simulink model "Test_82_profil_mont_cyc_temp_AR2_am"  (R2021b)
settings: Solver=FixedStepAuto  StartTime=0.0  StopTime=60*60*2
undefined symbols (not defined in the file): Ion, Lithium, Pe
libraries: fl_lib x31, nesl_utility x24, sdl_lib x11, simulink x5, simulink_extras x2, spsBatteryLib x1, spsCurrentVoltageSimscapeInterfaceLib x1, slpidlib x1, spspowerguiLib x1
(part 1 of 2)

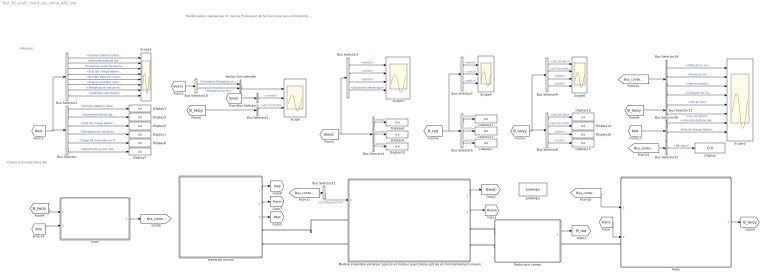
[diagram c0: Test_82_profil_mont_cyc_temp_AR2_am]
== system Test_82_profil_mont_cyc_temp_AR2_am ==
  note: Chaine d'énergie Twizy 80
  note: Modélisation réalisée par M. Garcia Professeur de S2I au lycée Louis Armand de Nogent sur Marne
  note: Mesures
  Batteries lithium : Subsystem  mask{Ubat_n=54, Qbat_n=105, Soc_init=100, Soc_min=10, T_amb=35, T_init=15, Nb_cycles=1000, Nb_charge_mensuelle=20, Nb_mois=25}
      mask prompts: Ubat_n "Tension nominale batterie en V"; Qbat_n "Capacité nominale en A.h"; Soc_init "Etat de charge initial"; Soc_min "Seuil minimum en %"; T_amb "Température ambiante extérieure en °C"; T_init "Température initiale du bloc batteries en °C"; Nb_cycles "Durée de vie batterie en nombre de cycles"; Nb_charge_mensuelle "Nombre de recharges mensuelles"; Nb_mois "Nombre de mois d'utilisation"
  Bus Selector : BusSelector  OutputSignals=tension batterie ubat(t),intensité batterie ibat(t),Etat de charge batterie soc(t) en %,Température cellule en °C,Capacité maximale en Ah,Nombre de cycles utilisés
  Bus Selector1 : BusSelector  OutputSignals=nm(t)
  Bus Selector10 : BusSelector  OutputSignals=Consigne fréquence en Hz,fréquence en Hz
  Bus Selector11 : BusSelector  OutputSignals=Consigne en %
  Bus Selector12 : BusSelector  OutputSignals=Nb_tour
  Bus Selector13 : BusSelector  OutputSignals=d(t) en km,v(t) en km/h
  Bus Selector14 : BusSelector  OutputSignals=Altitude en m,Pente en %,Vent en km/h,Consigne en %
  Bus Selector16 : BusSelector  OutputSignals=intensité batterie ibat(t),Etat de charge batterie soc(t) en %
  Bus Selector2 : BusSelector  OutputSignals=tension batterie ubat(t),intensité batterie ibat(t),Puissance consommée batterie pbat(t) en W,Etat de charge batterie soc(t) en %,Energie batterie consommée wbat_cons(t) en Wh,Energie batterie restante wbat_rest(t) en Wh,Température cellule en °C,Quadrant électrique
  Bus Selector3 : BusSelector  OutputSignals=v(t) en km/h
  Bus Selector4 : BusSelector  OutputSignals=nm(t),cm(t),pm(t)
  Bus Selector5 : BusSelector  OutputSignals=wm(t),cm(t),pm(t),Quadrant mécanique
  Bus Selector6 : BusSelector  OutputSignals=nr(t),cr(t),pr(t)
  Bus Selector7 : BusSelector  OutputSignals=wr(t),cr(t),pr(t)
  Bus Selector8 : BusSelector  OutputSignals=d(t) en km,v(t) en km/h,fm(t),pr(t)
  Bus Selector9 : BusSelector  OutputSignals=d(t) en km,v(t) en km/h,fm(t),pr(t)
  Display{,1..16} (17 alike) : Display
  Modele ensemble variateur Sevcon et moteur asynchrone Letrika en fonctionnement moyen : Subsystem  mask{Vbn=52, Tn=57, Nn=2100, fn=70, rend_mot=92, Jm=0.006, f_max_av=276, f_max_ar=41.7, rend_var=96, kp_n=1, ki_n=0.01, pas=0.1}
      mask prompts: Vbn "Tension bobinage nominale moteur en V"; Tn "Couple nominal en N.m"; Nn "Vitesse nominale moteur en tr/min"; fn "fréquence nominale moteur en Hz"; rend_mot "Rendement moteur en %"; Jm "Moment d'inertie moteur en kg.m²"; f_max_av "Fréquence maximale autorisée en marche avant en hz"; f_max_ar "Fréquence maximale autorisée en marche arrière en hz"; rend_var "Rendement variateur en %"; kp_n "Gain correcteur proportionnel"; ki_n "Gain correcteur intégral"; pas "Réglage pas solveur simscape"
  Profil : Subsystem  mask{Altitude_Pt_dep=307, Nb_portion=36, Pe_P=[4.2;6.7;5.6;5.9;6.8;7.2;6.5;6.1;7.4;3.7;3.6;8.4;7.2;8.4;6.6;4.2;3.9;0;-3.9;-4.2;-6.6;-8.4;-7.2;-8.4;-3.6;-3.7;-7.4;-6.1;-6.5;-7.2;-6.8;-5.9;-5.6;-6.7;-4.2;0], L_P=[1000;1000;1000;1000;1000;1000;1000;1000;1000;1000;1000;1000;1000;1000;1000;1000;400;2000;400;1000;1000;1000;1000;1000;1000;1000;1000;1000;1000;1000;1000;1000;1000;1000;1000;2000], Co_P=[50;50;50;50;50;50;50;50;50;50;50;50;50;50;50;50;50;25;60;60;60;60;60;60;60;60;60;60;60;60;60;60;60;60;60;25], Ve_P=[0;0;0;0;0;0;0;0;0;0;0;0;0;0;0;0;0;0;0;0;0;0;0;0;0;0;0;0;0;0;0;0;0;0;0;0], Nb_tour_max=2}
      mask prompts: Altitude_Pt_dep "Altitude du point de départ en m"; Nb_portion "Nombre de portion du circuit"; Pe_P "Pente des différentes portions en %"; L_P "Longueur des différentes portions en m"; Co_P "Consigne vitesse sur les différentes portions en %"; Ve_P "Vitesse du vent sur les différentes portions en km/h"; Nb_tour_max "Nombre de tour de circuit à parcourir"
  Reducteur comex : Subsystem  mask{ratio=(82*55)/(17*26), rend_red=96}
      mask prompts: ratio "Rapport de réduction"; rend_red "Rendement moyen transmission en %"
  Scope : Scope  NumInputPorts=3
  Scope1 : Scope  NumInputPorts=8
  Scope2 : Scope  NumInputPorts=8
  Scope3 : Scope  NumInputPorts=4
  Scope4 : Scope  NumInputPorts=3
  Scope5 : Scope  NumInputPorts=4
  Twizy : Subsystem  mask{n=2, a=733, b=955, h=900, S=1.33, Cx=0.64, M_twizy=403, M_cond=80, M_pass=0, M_Batt=71, t_jantes_av=13, l_pneu_av=125, h_broul_av=80, Prav=2.5, t_jantes_ar=13, l_pneu_ar=145, h_broul_ar=80, Prar=2.5}
      mask prompts: n "Nombre de roue par axe"; a "Distance entre position conducteur et l'axe de la roue avant en mm"; b "Distance entre position conducteur et l'axe de la roue arrière en mm"; h "Hauteur du centre de gravité passager en mm"; S "Surface frontale en m²"; Cx "Coefficient de trainée"; M_twizy "Masse twizy à vide en kg"; M_cond "Masse conducteur en kg"; M_pass "Masse passagers en kg"; M_Batt "Masse batteries en kg"; t_jantes_av "Taille jante en pouces"; l_pneu_av "Largeur en mm"; h_broul_av "Hauteur bande de roulement en %"; Prav "Pression pneus avant en bar"; t_jantes_ar "Taille jante en pouces"; l_pneu_ar "Largeur en mm"; h_broul_ar "Hauteur bande de roulement en %"; Prar "Pression pneus arrière en bar"
  Vector Concatenate : Concatenate
  powergui : spspowerguiLib/powergui  Priority=1  SimulationMode=Discrete  SampleTime=1  frequency=60  Iterations=50  frequencyindice=0  Pbase=100e6  ErrMax=1e-4  UnitsV=kV  UnitsW=MW  buscounter=0  FunctionMessages=off  echomessages=off  EnableUseOfTLC=off  CurrentSourceSwitches=off  DisableSnubberDevices=off  DisableRonSwitches=off  DisableVfSwitches=off  DisplayEquations=off  AutomaticDiscreteSolvers=off  SolverType=Tustin/Backward Euler (TBE)  Interpol=off  ExternalGateDelay=off  methode=off  Ts=100  x0status=blocks  SPID=on  SwTol=0  HookPort=off  NonlinearTolerance=1e-4  nMaxIteration=100  ContinueOnMaxIteration=off  RestoreLinks=warning  ResistiveCurrentMeasurement=off  Frange=[0:2:500]  Ylog=off  Xlog=on  ShowGrid=off  save=off  variable=ZData  structure=0  ZoomFFT=off  StartTime=0.0  cycles=1  DisplayStyle=1  fundamental=60  FreqAxis=off  MaxFrequency=1000  frequencyindicesteady=1  RmsSteady=1  display=off
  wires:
  Reducteur comex/1(Bus) -> [B_red]
  Twizy/1(Bus) -> [B_twizy]
  Modele ensemble variateur Sevcon et moteur asynchrone Letrika en fonctionnement moyen/1(Bus) -> [Bmot]
  [Freins] -> Twizy/2(Forces freinages avant et arrières)
  Modele ensemble variateur Sevcon et moteur asynchrone Letrika en fonctionnement moyen/2(Bus1) -> [Bvaria]
  Bus Selector11/1 -> Modele ensemble variateur Sevcon et moteur asynchrone Letrika en fonctionnement moyen/1(Consigne Accélérateur en %)  "<Consigne en %>"
  [B_twizy] -> Profil/1(Bus_Twizy)
  Profil/1(Contexte) -> [Bus_contexte]
  [Bus_contexte] -> Bus Selector11/1
  [Bus_contexte] -> Twizy/1(Contexte)
  Batteries lithium/1(Stop) -> [Stop]
  Batteries lithium/3(Bus batterie) -> [Bbat]
  Batteries lithium/2(Freinage) -> [Freins]
  [Stop] -> Profil/2(Stop)
  Bus Selector12/1 -> Display/1  "<Nb_tour>"
  [B_twizy] -> Bus Selector13/1
  [Bbat] -> Bus Selector16/1
  [Bvaria] -> Bus Selector10/1
  Bus Selector8/1 -> Display13/1  "<d(t) en km>"
  Bus Selector2/3 -> Scope1/3  "<Puissance consommée batterie pbat(t) en W>"
  Bus Selector/5 -> Display6/1  "<Capacité maximale en Ah>"
  [Bmot] -> Bus Selector4/1, Bus Selector5/1
  Bus Selector6/2 -> Display12/1  "<cr(t)>"
  Bus Selector6/1 -> Display11/1  "<nr(t)>"
  Bus Selector4/1 -> Display8/1  "<nm(t)>"
  Bus Selector9/3 -> Scope5/3  "<fm(t)>"
  Bus Selector5/3 -> Scope3/3  "<pm(t)>"
  Bus Selector/3 -> Display5/1  "<Etat de charge batterie soc(t) en %>"
  Bus Selector14/3 -> Scope2/3  "<Vent en km/h>"
  Bus Selector13/2 -> Scope2/6  "<v(t) en km/h>"
  [Bbat] -> Bus Selector2/1, Bus Selector/1
  Bus Selector2/8 -> Scope1/8  "<Quadrant électrique>"
  [B_twizy] -> Bus Selector3/1
  Bus Selector7/2 -> Scope4/2  "<cr(t)>"
  Bus Selector7/1 -> Scope4/1  "<wr(t)>"
  Bus Selector1/1 -> Scope/2  "<nm(t)>"
  Bus Selector7/3 -> Scope4/3  "<pr(t)>"
  Bus Selector/1 -> Display3/1  "<tension batterie ubat(t)>"
  Bus Selector2/1 -> Scope1/1  "<tension batterie ubat(t)>"
  Bus Selector/4 -> Display1/1  "<Température cellule en °C>"
  Bus Selector/2 -> Display4/1  "<intensité batterie ibat(t)>"
  Bus Selector14/2 -> Scope2/2  "<Pente en %>"
  Bus Selector5/1 -> Scope3/1  "<wm(t)>"
  Bus Selector14/4 -> Scope2/4  "<Consigne en %>"
  Bus Selector4/2 -> Display9/1  "<cm(t)>"
  Bus Selector2/5 -> Scope1/5  "<Energie batterie consommée wbat_cons(t) en Wh>"
  [B_twizy] -> Bus Selector9/1, Bus Selector8/1
  Bus Selector2/2 -> Scope1/2  "<intensité batterie ibat(t)>"
  Bus Selector10/2 -> Vector Concatenate/2  "<fréquence en Hz>"
  Bus Selector13/1 -> Scope2/5  "<d(t) en km>"
  Bus Selector/6 -> Display7/1  "<Nombre de cycles utilisés>"
  Bus Selector9/4 -> Scope5/4  "<pr(t)>"
  Bus Selector10/1 -> Vector Concatenate/1  "<Consigne fréquence en Hz>"
  Bus Selector14/1 -> Scope2/1  "<Altitude en m>"
  Bus Selector9/2 -> Scope5/2  "<v(t) en km/h>"
  Bus Selector16/2 -> Scope2/8  "<Etat de charge batterie soc(t) en %>"
  Bus Selector9/1 -> Scope5/1  "<d(t) en km>"
  Bus Selector5/2 -> Scope3/2  "<cm(t)>"
  Bus Selector5/4 -> Scope3/4  "<Quadrant mécanique>"
  [Bmot] -> Bus Selector1/1
  Bus Selector8/2 -> Display14/1  "<v(t) en km/h>"
  Bus Selector2/6 -> Scope1/6  "<Energie batterie restante wbat_rest(t) en Wh>"
  Bus Selector8/3 -> Display16/1  "<fm(t)>"
  Bus Selector3/1 -> Scope/3  "<v(t) en km/h>"
  Bus Selector6/3 -> Display2/1  "<pr(t)>"
  [Bus_contexte] -> Bus Selector14/1
  Bus Selector4/3 -> Display10/1  "<pm(t)>"
  Vector Concatenate/1 -> Scope/1
  Bus Selector8/4 -> Display15/1  "<pr(t)>"
  Bus Selector16/1 -> Scope2/7  "<intensité batterie ibat(t)>"
  Bus Selector2/7 -> Scope1/7  "<Température cellule en °C>"
  [B_red] -> Bus Selector7/1, Bus Selector6/1
  Bus Selector2/4 -> Scope1/4  "<Etat de charge batterie soc(t) en %>"
  [Bus_contexte] -> Bus Selector12/1
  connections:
  Reducteur comex/RConn1 -- Twizy/LConn1
  Reducteur comex/LConn2 -- Modele ensemble variateur Sevcon et moteur asynchrone Letrika en fonctionnement moyen/RConn2
  Reducteur comex/LConn1 -- Modele ensemble variateur Sevcon et moteur asynchrone Letrika en fonctionnement moyen/RConn1
  Modele ensemble variateur Sevcon et moteur asynchrone Letrika en fonctionnement moyen/LConn2 -- Batteries lithium/RConn2
  Modele ensemble variateur Sevcon et moteur asynchrone Letrika en fonctionnement moyen/LConn1 -- Batteries lithium/RConn1

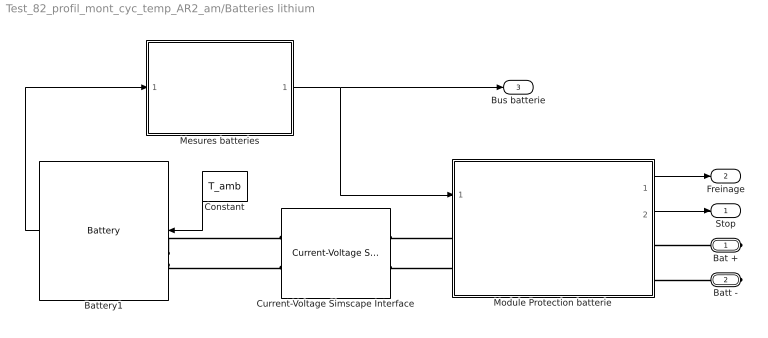
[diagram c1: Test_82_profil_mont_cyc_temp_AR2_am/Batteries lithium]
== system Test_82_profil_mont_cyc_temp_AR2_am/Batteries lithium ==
  Battery1 : spsBatteryLib/Battery  BatType=Lithium-Ion  ShowTempParam=on  ThermalPreset=no  ShowAgeParam=on  NomV=Ubat_n  NomQ=Qbat_n  SOC=Soc_init  Batt_Tr=30  PresetModel=on  MaxQ=105  MinV=40.5  FullV=62.8553  Dis_rate=45.6522  R=0.0051429  Normal_OP=94.9565  expZone="[58.3408       5.1587]"  current=[100 150 200]  Units=Time  Tci=T_init  NomT=25  T2=0  MaxQ2=Qbat_n/1.1517  FullV2=1.1933*Ubat_n  Normal_OP2=Ubat_n/1.1576  expZone2=[1.1338*Ubat_n Qbat_n/61]  Rca=0.06  ti=1000  Dp=0  Neq0=Nb_charge_mensuelle*Nb_mois  Tsim=30  Ta1=23  Qeol=0.9*Qbat_n  Reol=0.0126*1.2  Char_age=[0.38*Qbat_n, 0.495*Qbat_n]  Dis_age=[0.38*Qbat_n, 2*Qbat_n]  N1=Nb_cycles  N2=7*Nb_cycles  N3=Nb_cycles/1.5  N4=Nb_cycles*0.9733  Ta2=45  N5=Nb_cycles*0.655
  Constant : Constant  Value=T_amb
  Current-Voltage Simscape Interface : spsCurrentVoltageSimscapeInterfaceLib/Current-Voltage Simscape Interface  DFT=off  FMode=Unit delay (discrete)  T=1e-6  Ts=-1  i0=0  v0=52  Sd=Simscape side  Measurements=off
  Mesures batteries : Subsystem
  Module Protection batterie : Subsystem
  Bat + : PMIOPort  Side=Right
  Batt - : PMIOPort  Port=2  Side=Right
  Stop : Outport  VectorParamsAs1DForOutWhenUnconnected=off
  Freinage : Outport  Port=2  VectorParamsAs1DForOutWhenUnconnected=off
  Bus batterie : Outport  Port=3  VectorParamsAs1DForOutWhenUnconnected=off
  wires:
  Battery1/1 -> Mesures batteries/1(Bus batteries)
  Mesures batteries/1(Bus_ batteries) -> Module Protection batterie/1(Bus batterie), Bus batterie/1
  Module Protection batterie/1(Freinage) -> Freinage/1
  Module Protection batterie/2(Stop) -> Stop/1
  Constant/1 -> Battery1/1
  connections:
  Battery1/LConn2 -- Current-Voltage Simscape Interface/LConn2
  Battery1/LConn1 -- Current-Voltage Simscape Interface/LConn1
  Module Protection batterie/RConn2 -- Batt -/RConn1
  Module Protection batterie/RConn1 -- Bat +/RConn1
  Module Protection batterie/LConn1 -- Current-Voltage Simscape Interface/RConn1
  Module Protection batterie/LConn2 -- Current-Voltage Simscape Interface/RConn2

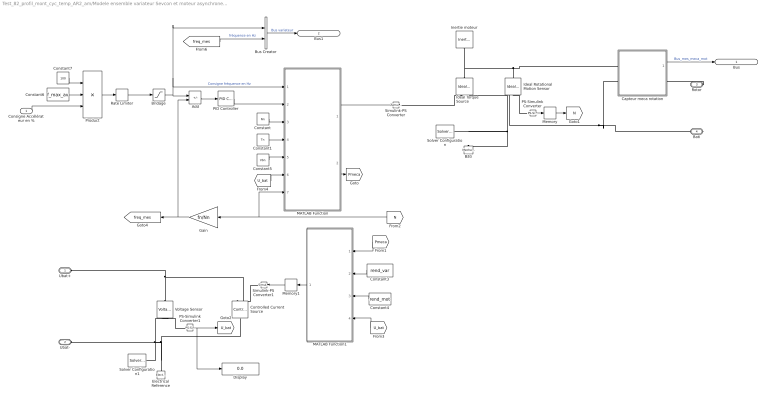
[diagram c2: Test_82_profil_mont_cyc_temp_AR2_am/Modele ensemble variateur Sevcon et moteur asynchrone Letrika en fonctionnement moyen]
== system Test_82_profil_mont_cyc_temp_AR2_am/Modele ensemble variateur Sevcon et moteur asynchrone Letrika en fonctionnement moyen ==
  Consigne Accélérateur en % : Inport
  Add : Sum  Inputs=+-
  Bridage : Saturate  UpperLimit=f_max_av  LowerLimit=-f_max_ar
  Bus Creator : BusCreator  Inputs=2
  Bâti : fl_lib/Mechanical/Rotational Elements/Mechanical Rotational Reference
  Capteur meca rotation : Subsystem
  Constant : Constant  Value=Nn
  Constant1 : Constant  Value=Tn
  Constant3 : Constant  Value=rend_var
  Constant4 : Constant  Value=rend_mot
  Constant5 : Constant  Value=Vbn
  Constant6 : Constant  Value=f_max_av
  Constant7 : Constant  Value=100
  Controlled Current Source : fl_lib/Electrical/Electrical Sources/Controlled Current Source
  Display : Display
  Electrical Reference : fl_lib/Electrical/Electrical Elements/Electrical Reference
  Gain : Gain  Gain=fn/Nn
  Ideal Rotational Motion Sensor : fl_lib/Mechanical/Mechanical Sensors/Ideal Rotational Motion Sensor  wrap_angle=simscape.enum.onoff.off  offset=0 rad
  Ideal Torque Source : fl_lib/Mechanical/Mechanical Sources/Ideal Torque Source
  Inertie moteur : fl_lib/Mechanical/Rotational Elements/Inertia  inertia=Jm kg*m^2  num_ports=foundation.enum.numPorts2.one  w_specify=off  w_priority=High  w=0 rad/s  w_nominal_specify=off  w_nominal_unit=rad/s  w_nominal_value=1  t_specify=off  t_priority=None  t=0 N*m  t_nominal_specify=off  t_nominal_unit=N*m  t_nominal_value=1
  MATLAB Function : MATLAB Function  TreatAsAtomicUnit=on
  MATLAB Function1 : MATLAB Function  TreatAsAtomicUnit=on
  Memory : Memory
  Memory1 : Memory
  PID Controller : slpidlib/PID Controller  Controller=PID  Form=Parallel  TimeDomain=Continuous-time  UseExternalTs=off  SampleTime=-1  IntegratorMethod=Forward Euler  FilterMethod=Forward Euler  ControllerParametersSource=internal  P=kp_n  I=ki_n  D=0  UseFilter=on  N=100  TunerSelectOption=Transfer Function Based (PID Tuner App)  InitialConditionSource=internal  InitialConditionForIntegrator=0  InitialConditionForFilter=0  DifferentiatorICPrevScaledInput=0  ExternalReset=none  TrackingMode=off  Kt=1  LimitOutput=off  SatLimitsSource=internal  UpperSaturationLimit=inf  LowerSaturationLimit=-inf  LinearizeAsGain=on  AntiWindupMode=none  Kb=1  POutMin=[]  POutMax=[]  IOutMin=[]  IOutMax=[]  DOutMin=[]  DOutMax=[]  NOutMin=[]  NOutMax=[]  SumOutMin=[]  SumOutMax=[]  SaturationOutMin=[]  SaturationOutMax=[]  PParamMin=[]  PParamMax=[]  IParamMin=[]  IParamMax=[]  DParamMin=[]  DParamMax=[]  NParamMin=[]  NParamMax=[]  KbParamMin=[]  KbParamMax=[]  KtParamMin=[]  KtParamMax=[]  KbOutMin=[]  KbOutMax=[]  KtOutMin=[]  KtOutMax=[]  IntegratorOutMin=[]  IntegratorOutMax=[]  FilterOutMin=[]  FilterOutMax=[]  SumI1OutMin=[]  SumI1OutMax=[]  SumI2OutMin=[]  SumI2OutMax=[]  SumI3OutMin=[]  SumI3OutMax=[]  SumI4OutMin=[]  SumI4OutMax=[]  SumDOutMin=[]  SumDOutMax=[]  DifferentiatorOutMin=[]  DifferentiatorOutMax=[]  FilterDiffOutCoefMin=[]  FilterDiffOutCoefMax=[]  ReciprocalOutMin=[]  ReciprocalOutMax=[]  SumDenOutMin=[]  SumDenOutMax=[]  SumNumOutMin=[]  SumNumOutMax=[]  DivideOutMin=[]  DivideOutMax=[]  UdiffTsProdOutMin=[]  UdiffTsProdOutMax=[]  NTsProdOutMin=[]  NTsProdOutMax=[]  UintegralTsProdOutMin=[]  UintegralTsProdOutMax=[]  UngainTsProdOutMin=[]  UngainTsProdOutMax=[]  IntegratorContinuousStateAttributes=''  IntegratorStateMustResolveToSignalObject=off  IntegratorRTWStateStorageClass=Auto  FilterContinuousStateAttributes=''  FilterStateMustResolveToSignalObject=off  FilterRTWStateStorageClass=Auto  ParallelPVariant=InternalParameters  IdealPVariant=Disabled  IVariant=InternalParameters  DVariant=InternalParameters  IntegratorVariant=Continuous  SatVariant=Disabled  AWVariant=Passthrough  PCopyVariant=Disabled  TRVariant=Disabled  FdbkBlocksVariant=Forward  IdealPFdbkVariant=Disabled  SatFdbkVariant=Disabled  DerivativeFilterVariant=ContFilter  NVariant=InternalParameters  NCopyVariant=Disabled  FilterICVariant=InternalICsFilter  IntegratorICVariant=InternalICs  ExternalResetVariant=Disabled  TRSumVariant=Passthrough  SumFdbkVariant=Disabled  SumVariant=Sum_PID  TsampFilterVariant=InternalTs  TsampNgainVariant=Passthrough  TsampIntegralVariant=Passthrough  ExternalSaturationOutDataTypeStr=Inherit: Same as second input
  PS-Simulink Converter : nesl_utility/PS-Simulink Converter  PhysicalDomain=network_engine_domain  SubClassName=ps_output  LeftPortType=input  RightPortType=output  PseudoPeriodic=off  Frequencies=[]  Unit=rpm  AffineConversion=off
  PS-Simulink Converter1 : nesl_utility/PS-Simulink Converter  PhysicalDomain=network_engine_domain  SubClassName=ps_output  LeftPortType=input  RightPortType=output  PseudoPeriodic=off  Frequencies=[]  Unit=V  AffineConversion=off
  Product : Product  Inputs=/**
  Rate Limiter : RateLimiter  RisingSlewLimit=80  FallingSlewLimit=-inf  SampleTimeMode=inherited
  Simulink-PS Converter : nesl_utility/Simulink-PS Converter  PhysicalDomain=network_engine_domain  SubClassName=ps_input  LeftPortType=input  RightPortType=output  PseudoPeriodic=off  Frequencies=[]  NoiseDistribution=none  NoiseParameters=[]  Unit=N*m  AffineConversion=off  FilteringAndDerivatives=provide  SimscapeFilterOrder=1  InputFilterTimeConstant=0.001  UdotUserProvided=0
  Simulink-PS Converter1 : nesl_utility/Simulink-PS Converter  PhysicalDomain=network_engine_domain  SubClassName=ps_input  LeftPortType=input  RightPortType=output  PseudoPeriodic=off  Frequencies=[]  NoiseDistribution=none  NoiseParameters=[]  Unit=A  AffineConversion=off  FilteringAndDerivatives=provide  SimscapeFilterOrder=1  InputFilterTimeConstant=0.001  UdotUserProvided=0
  Solver Configuration : nesl_utility/Solver Configuration  PhysicalDomain=network_engine_domain  SubClassName=solver  LeftPortType=input  RightPortType=generic  Tones=[]  Harmonics=[]  SimulateNoise=off  Profile=off  UseLocalSampling=off  EnableSwitchedLinearOptims=on  FrequencyDomain=off  UseCCode=off  RelTol=0.001  AbsTol=1e-06  MinStep=1e-09  ToWorkspace=off  RevertToSquareIcSolve=off  NumHomotopyIterations=100  PhasorMode=off  PhasorModeNumHarmonics=1  DoDC=off  ResidualTolerance=1e-9  UseLocalSolver=on  LocalSolverChoice=NE_BACKWARD_EULER_ADVANCER  LocalSolverSampleTime=pas  DoFixedCost=on  MaxNonlinIter=3  MaxModeIter=2  ComputeImpulses=off  ImpulseIterations=2  LinearAlgebra=auto  EquationFormulation=NE_TIME_EF  DelaysMemoryBudget=1024  AutomaticFiltering=on  FilteringTimeConstant=0.001  PartitionStorageMethod=AS_NEEDED  PartitionMemoryBudget=1024  PartitionMethod=FAST
  Solver Configuration1 : nesl_utility/Solver Configuration  PhysicalDomain=network_engine_domain  SubClassName=solver  LeftPortType=input  RightPortType=generic  Tones=[]  Harmonics=[]  SimulateNoise=off  Profile=off  UseLocalSampling=off  EnableSwitchedLinearOptims=on  FrequencyDomain=off  UseCCode=off  RelTol=0.001  AbsTol=1e-06  MinStep=1e-09  ToWorkspace=off  RevertToSquareIcSolve=off  NumHomotopyIterations=100  PhasorMode=off  PhasorModeNumHarmonics=1  DoDC=off  ResidualTolerance=1e-9  UseLocalSolver=on  LocalSolverChoice=NE_BACKWARD_EULER_ADVANCER  LocalSolverSampleTime=pas  DoFixedCost=on  MaxNonlinIter=3  MaxModeIter=2  ComputeImpulses=off  ImpulseIterations=2  LinearAlgebra=auto  EquationFormulation=NE_TIME_EF  DelaysMemoryBudget=1024  AutomaticFiltering=on  FilteringTimeConstant=0.001  PartitionStorageMethod=AS_NEEDED  PartitionMemoryBudget=1024  PartitionMethod=FAST
  Voltage Sensor : fl_lib/Electrical/Electrical Sensors/Voltage Sensor
  Ubat+ : PMIOPort  Side=Left
  Ubat- : PMIOPort  Port=2  Side=Left
  Rotor : PMIOPort  Port=3  Side=Right
  Bati : PMIOPort  Port=4  Side=Right
  Bus : Outport  VectorParamsAs1DForOutWhenUnconnected=off
  Bus1 : Outport  Port=2  VectorParamsAs1DForOutWhenUnconnected=off
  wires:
  Capteur meca rotation/1(Out6) -> Bus/1  "Bus_mes_meca_mot"
  PS-Simulink Converter/1 -> Memory/1
  Constant/1 -> MATLAB Function/3(Nn)
  Constant1/1 -> MATLAB Function/4(Tn)
  [N] -> Gain/1, MATLAB Function/7(Nmes)
  Add/1 -> PID Controller/1
  PID Controller/1 -> MATLAB Function/2(T_in)
  Consigne Accélérateur en %/1 -> Product/3
  Memory/1 -> [N]
  MATLAB Function1/1(I_bat) -> Memory1/1
  MATLAB Function/2(P_meca) -> [Pmeca]
  [Pmeca] -> MATLAB Function1/1(Pmeca)
  Constant3/1 -> MATLAB Function1/2(rend_var)
  Constant4/1 -> MATLAB Function1/3(rend_mot)
  PS-Simulink Converter1/1 -> Display/1, [U_bat]
  [U_bat] -> MATLAB Function1/4(U_bat)
  [U_bat] -> MATLAB Function/6(U_bat)
  Constant5/1 -> MATLAB Function/5(Un)
  Gain/1 -> [freq_mes], Add/2
  Constant6/1 -> Product/2
  Constant7/1 -> Product/1
  Bus Creator/1 -> Bus1/1  "Bus variateur"
  Bridage/1 -> Bus Creator/1, MATLAB Function/1(Consigne_frequence), Add/1  "Consigne fréquence en Hz"
  [freq_mes] -> Bus Creator/2  "fréquence en Hz"
  Memory1/1 -> Simulink-PS Converter1/1
  MATLAB Function/1(T_out) -> Simulink-PS Converter/1
  Product/1 -> Rate Limiter/1
  Rate Limiter/1 -> Bridage/1
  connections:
  Rotor/RConn1 -- Capteur meca rotation/RConn1
  Ideal Rotational Motion Sensor/RConn1 -- Bâti/LConn1 -- Solver Configuration/RConn1 -- Ideal Torque Source/RConn2 -- Bati/RConn1 -- Capteur meca rotation/LConn2
  Ideal Torque Source/LConn1 -- Inertie moteur/LConn1 -- Capteur meca rotation/LConn1 -- Ideal Rotational Motion Sensor/LConn1
  PS-Simulink Converter/LConn1 -- Ideal Rotational Motion Sensor/RConn2
  Simulink-PS Converter/RConn1 -- Ideal Torque Source/RConn1
  Ubat-/RConn1 -- Controlled Current Source/LConn1 -- Electrical Reference/LConn1 -- Solver Configuration1/RConn1 -- Voltage Sensor/RConn2
  PS-Simulink Converter1/LConn1 -- Voltage Sensor/RConn1
  Simulink-PS Converter1/RConn1 -- Controlled Current Source/RConn1
  Voltage Sensor/LConn1 -- Ubat+/RConn1 -- Controlled Current Source/RConn2

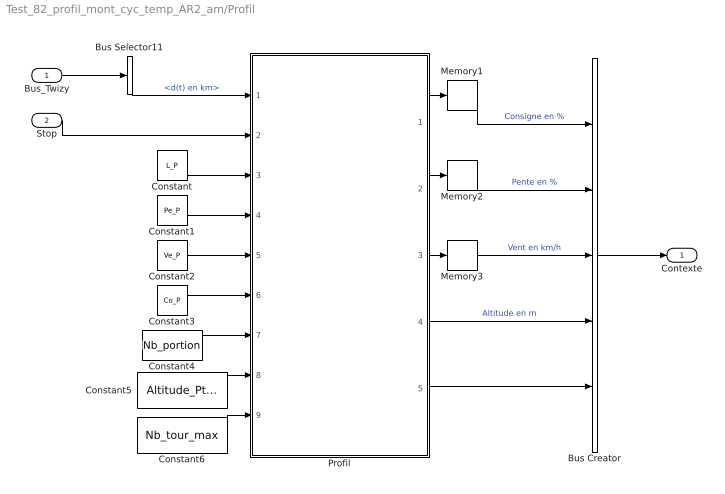
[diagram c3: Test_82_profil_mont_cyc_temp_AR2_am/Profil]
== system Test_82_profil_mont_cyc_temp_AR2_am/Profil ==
  Bus_Twizy : Inport
  Stop : Inport  Port=2
  Bus Creator : BusCreator  Inputs=5
  Bus Selector11 : BusSelector  OutputSignals=d(t) en km
  Constant : Constant  Value=L_P
  Constant1 : Constant  Value=Pe_P
  Constant2 : Constant  Value=Ve_P
  Constant3 : Constant  Value=Co_P
  Constant4 : Constant  Value=Nb_portion
  Constant5 : Constant  Value=Altitude_Pt_dep
  Constant6 : Constant  Value=Nb_tour_max
  Memory1 : Memory
  Memory2 : Memory
  Memory3 : Memory
  Profil : Stateflow chart  TreatAsAtomicUnit=on
  Contexte : Outport  VectorParamsAs1DForOutWhenUnconnected=off
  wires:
  Profil/3(Vent) -> Memory3/1
  Profil/4(Hauteur) -> Bus Creator/4  "Altitude en m"
  Constant/1 -> Profil/3(L_P)
  Constant6/1 -> Profil/9(Nb_tour_max)
  Constant5/1 -> Profil/8(Altitude_Pt_dep)
  Constant3/1 -> Profil/6(Co_P)
  Constant4/1 -> Profil/7(Nb_portion)
  Constant2/1 -> Profil/5(Ve_P)
  Bus_Twizy/1 -> Bus Selector11/1
  Constant1/1 -> Profil/4(Pe_P)
  Memory1/1 -> Bus Creator/1  "Consigne en %"
  Stop/1 -> Profil/2(Stop)
  Profil/2(Pente) -> Memory2/1
  Memory3/1 -> Bus Creator/3  "Vent en km/h"
  Memory2/1 -> Bus Creator/2  "Pente en %"
  Profil/1(Consigne_vit) -> Memory1/1
  Bus Selector11/1 -> Profil/1(position)  "<d(t) en km>"
  Bus Creator/1 -> Contexte/1
  Profil/5(Nb_tour) -> Bus Creator/5

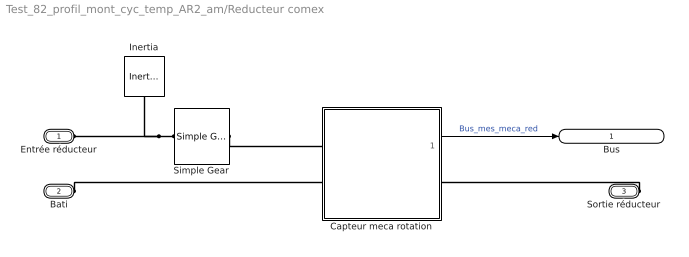
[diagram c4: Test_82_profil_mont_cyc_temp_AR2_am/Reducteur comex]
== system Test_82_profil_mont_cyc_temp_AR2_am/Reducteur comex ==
  Capteur meca rotation : Subsystem
  Inertia : fl_lib/Mechanical/Rotational Elements/Inertia  inertia=0.0725 kg*m^2  num_ports=foundation.enum.numPorts2.one  w_specify=off  w_priority=High  w=0 rad/s  w_nominal_specify=off  w_nominal_unit=rad/s  w_nominal_value=1  t_specify=off  t_priority=None  t=0 N*m  t_nominal_specify=off  t_nominal_unit=N*m  t_nominal_value=1
  Simple Gear : sdl_lib/Gears/Simple Gear  ratio=ratio  rotation_direction=3-2*(1)  friction_model=2  T_noload=0.1 N*m  T_nom=5 N*m  efficiency_nom=0.8  efficiency=rend_red/100  temperature_TLU=[280, 300, 320] K  load_TLU=[1, 5, 10] N*m  efficiency_TLU=[.95, .9, .85]  efficiency_TLU2=[.85, .8, .75; .95, .9, .85; .85, .8, .7]  w_thr=0.01 rad/s  pwr_thr=0.001 W  backlash_model=sdl.enum.backlashModel.Off  backlash_distance=1e-3 mm  x0=0 mm  r_base=0.1 m  hardstop_model=simscape.enum.hardstop.smooth  transition=1e-4 mm  backlash_stiffness=1e7 N/m  backlash_damping=1e6 N*s/m  e=0  v_tol=0.001 m/s  mu_visc=[0, 0] N*m/(rad/s)  enable_faults=0  efficiency_fault=0.05  external_fault=simscape.enum.onoff.off  temporal_fault=0  fault_time=5 s  fault_angles=pi / 12 rad  report_fault=(1)-1  thermal_mass=50 J/K  temperature_specify=off  temperature_priority=High  temperature=300 K  temperature_nominal_specify=off  temperature_nominal_unit=K  temperature_nominal_value=1  x_backlash_specify=off  x_backlash_priority=None  x_backlash=0 mm  x_backlash_nominal_specify=off  x_backlash_nominal_unit=mm  x_backlash_nominal_value=1  f_hardstop_specify=off  f_hardstop_priority=None  f_hardstop=0 N  f_hardstop_nominal_specify=off  f_hardstop_nominal_unit=N  f_hardstop_nominal_value=1  v_backlash_specify=off  v_backlash_priority=None  v_backlash=0 m/s  v_backlash_nominal_specify=off  v_backlash_nominal_unit=m/s  v_backlash_nominal_value=1
  Entrée réducteur : PMIOPort  Side=Left
  Bati : PMIOPort  Port=2  Side=Left
  Sortie réducteur : PMIOPort  Port=3  Side=Right
  Bus : Outport  VectorParamsAs1DForOutWhenUnconnected=off
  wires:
  Capteur meca rotation/1(Out6) -> Bus/1  "Bus_mes_meca_red"
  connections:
  Sortie réducteur/RConn1 -- Capteur meca rotation/RConn1
  Simple Gear/LConn1 -- Inertia/LConn1 -- Entrée réducteur/RConn1
  Bati/RConn1 -- Capteur meca rotation/LConn2
  Simple Gear/RConn1 -- Capteur meca rotation/LConn1

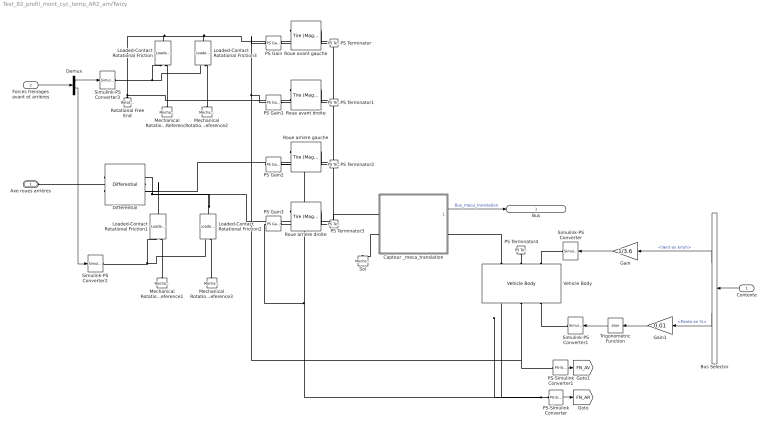
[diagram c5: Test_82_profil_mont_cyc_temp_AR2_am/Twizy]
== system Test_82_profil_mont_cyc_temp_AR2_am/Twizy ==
  Contexte : Inport
  Forces freinages avant et arrières : Inport  Port=2
  Bus Selector : BusSelector  OutputSignals=Vent en km/h,Pente en %
  Capteur _meca_translation : Subsystem
  Demux : Demux  Outputs=2
  Differential : sdl_lib/Gears/Differential  driveshaft_location=2  cd_ratio=1  friction_model=1  efficiency=[ 0.85 0.92 ]  temperature_TLU=[280, 300, 320] K  efficiency_ss_TLU=[.95, .9, .85]  efficiency_cd_TLU=[.95, .9, .85]  pwr_thr=[.001, .001] W  mu_visc=[ 0 0 ] N*m/(rad/s)  model_inertia=1  carrier_inertia=0.2 kg*m^2  planet_inertia=0.02 kg*m^2  thermal_mass=50 J/K  T_init=300 K
  Gain : Gain  Gain=1/3.6
  Gain1 : Gain  Gain=0.01
  Loaded-Contact Rotational Friction : sdl_lib/Brakes & Detents/Rotational/Loaded-Contact Rotational Friction  geometry_model=1  r_eff=280 mm  d_o=150 mm  d_i=100 mm  friction_model=1  mu_w_vector=[ 0 0.1 0.2 0.3 0.4 0.5 1 2 5 10 100 1000 ] rad/s  temperature_TLU=[280, 300, 320] K  mu_static=0.35  mu_static_vector=[.4, .38, .36]  mu_coulomb=0.3  mu_coulomb_vector=[ 0.29 0.28 0.26 0.22 0.21 0.2 0.2 0.19 0.19 0.19 0.19 0.19 ]  mu_coulomb_temp_vector=[.3, .28, .25]  mu_coulomb_matrix=[.34, .32, .3; .3, .28, .25; .25, .2, .15]  mu_interp_method=simscape.enum.interpolation.linear  mu_extrap_method=simscape.enum.extrapolation.linear  w_tol=0.001 rad/s  force_min=1 N  mu_visc=0 N*m/(rad/s)  initial_state_locked=0  enable_faults=simscape.enum.onoff.off  fault_type=sdl.enum.clutchFault.lock  external_fault=simscape.enum.onoff.off  temporal_fault=simscape.enum.onoff.off  fault_time=5 s  report_fault=simscape.enum.assert.action.none  thermal_mass=50 kJ/K  T_init=300 K
  Loaded-Contact Rotational Friction1 : sdl_lib/Brakes & Detents/Rotational/Loaded-Contact Rotational Friction  geometry_model=1  r_eff=280 mm  d_o=150 mm  d_i=100 mm  friction_model=1  mu_w_vector=[ 0 0.1 0.2 0.3 0.4 0.5 1 2 5 10 100 1000 ] rad/s  temperature_TLU=[280, 300, 320] K  mu_static=0.35  mu_static_vector=[.4, .38, .36]  mu_coulomb=0.3  mu_coulomb_vector=[ 0.29 0.28 0.26 0.22 0.21 0.2 0.2 0.19 0.19 0.19 0.19 0.19 ]  mu_coulomb_temp_vector=[.3, .28, .25]  mu_coulomb_matrix=[.34, .32, .3; .3, .28, .25; .25, .2, .15]  mu_interp_method=1  mu_extrap_method=1  w_tol=0.001 rad/s  force_min=1 N  mu_visc=0 N*m/(rad/s)  initial_state_locked=0  enable_faults=simscape.enum.onoff.off  fault_type=sdl.enum.clutchFault.lock  external_fault=simscape.enum.onoff.off  temporal_fault=simscape.enum.onoff.off  fault_time=5 s  report_fault=simscape.enum.assert.action.none  thermal_mass=50 kJ/K  T_init=300 K
  Loaded-Contact Rotational Friction2 : sdl_lib/Brakes & Detents/Rotational/Loaded-Contact Rotational Friction  geometry_model=1  r_eff=280 mm  d_o=150 mm  d_i=100 mm  friction_model=1  mu_w_vector=[ 0 0.1 0.2 0.3 0.4 0.5 1 2 5 10 100 1000 ] rad/s  temperature_TLU=[280, 300, 320] K  mu_static=0.35  mu_static_vector=[.4, .38, .36]  mu_coulomb=0.3  mu_coulomb_vector=[ 0.29 0.28 0.26 0.22 0.21 0.2 0.2 0.19 0.19 0.19 0.19 0.19 ]  mu_coulomb_temp_vector=[.3, .28, .25]  mu_coulomb_matrix=[.34, .32, .3; .3, .28, .25; .25, .2, .15]  mu_interp_method=1  mu_extrap_method=1  w_tol=0.001 rad/s  force_min=1 N  mu_visc=0 N*m/(rad/s)  initial_state_locked=0  enable_faults=simscape.enum.onoff.off  fault_type=sdl.enum.clutchFault.lock  external_fault=simscape.enum.onoff.off  temporal_fault=simscape.enum.onoff.off  fault_time=5 s  report_fault=simscape.enum.assert.action.none  thermal_mass=50 kJ/K  T_init=300 K
  Loaded-Contact Rotational Friction3 : sdl_lib/Brakes & Detents/Rotational/Loaded-Contact Rotational Friction  geometry_model=1  r_eff=280 mm  d_o=150 mm  d_i=100 mm  friction_model=1  mu_w_vector=[ 0 0.1 0.2 0.3 0.4 0.5 1 2 5 10 100 1000 ] rad/s  temperature_TLU=[280, 300, 320] K  mu_static=0.35  mu_static_vector=[.4, .38, .36]  mu_coulomb=0.3  mu_coulomb_vector=[ 0.29 0.28 0.26 0.22 0.21 0.2 0.2 0.19 0.19 0.19 0.19 0.19 ]  mu_coulomb_temp_vector=[.3, .28, .25]  mu_coulomb_matrix=[.34, .32, .3; .3, .28, .25; .25, .2, .15]  mu_interp_method=simscape.enum.interpolation.linear  mu_extrap_method=simscape.enum.extrapolation.linear  w_tol=0.001 rad/s  force_min=1 N  mu_visc=0 N*m/(rad/s)  initial_state_locked=0  enable_faults=simscape.enum.onoff.off  fault_type=sdl.enum.clutchFault.lock  external_fault=simscape.enum.onoff.off  temporal_fault=simscape.enum.onoff.off  fault_time=5 s  report_fault=simscape.enum.assert.action.none  thermal_mass=50 kJ/K  T_init=300 K
  Mechanical Rotational Reference{,1..3} (4 alike) : fl_lib/Mechanical/Rotational Elements/Mechanical Rotational Reference
  PS Gain{,1..3} (4 alike) : fl_lib/Physical Signals/Functions/PS Gain  gain=0.5
  PS Terminator{,1..4} (5 alike) : fl_lib/Physical Signals/Sinks/PS Terminator
  PS-Simulink Converter : nesl_utility/PS-Simulink Converter  PhysicalDomain=network_engine_domain  SubClassName=ps_output  LeftPortType=input  RightPortType=output  PseudoPeriodic=off  Frequencies=[]  Unit=N  AffineConversion=off
  PS-Simulink Converter1 : nesl_utility/PS-Simulink Converter  PhysicalDomain=network_engine_domain  SubClassName=ps_output  LeftPortType=input  RightPortType=output  PseudoPeriodic=off  Frequencies=[]  Unit=N  AffineConversion=off
  Rotational Free End : fl_lib/Mechanical/Rotational Elements/Rotational Free End  w_specify=off  w_priority=None  w=0 rad/s  w_nominal_specify=off  w_nominal_unit=rad/s  w_nominal_value=1
  Roue arriere droite : sdl_lib/Tires & Vehicles/Tire (Magic Formula)  parameterization=sdl.enum.magic_tire_model.constant  F_z1=3e+3 N  F_x1=3.5e+3 N  kappa1=10  B_m=10  C_m=1.9  D_m=1  E_m=0.97  fz0=4e+3 N  p_Cx=1.685  p_Dx=[ 1.21 -0.037 ]  p_Ex=[ 0.344 0.095 -0.02 0 ]  p_Kx=[ 21.51 -0.163 0.245 ]  p_Hx=[ -0.002 0.002 ]  p_Vx=[ 0 0 ]  r_e=(t_jantes_av*25.4+2*l_pneu_av*h_broul_av/100)/2 mm  model_compliance=sdl.enum.compliance.on  stiffness=1e+6 N/m  damping=1000 N/(m/s)  model_inertia=sdl.enum.model_inertia.on  inertia=0.12 kg*m^2  initial_velocity=0 rad/s  model_resistance=simscape.enum.onoff.on  resistance_model=sdl.enum.rollingResistanceParameterization.velocity  coeff=0.027*Pe  p_tire=Prar bar  alpha=-0.003  beta=0.76  coeff_a=84e-4  coeff_b=6.2e-4 s/m  coeff_c=1.6e-4 s^2/m^2  v_thr=1e-3 m/s  v_tr_thr=0.1 m/s
  Roue arriere gauche : sdl_lib/Tires & Vehicles/Tire (Magic Formula)  parameterization=sdl.enum.magic_tire_model.constant  F_z1=3e+3 N  F_x1=3.5e+3 N  kappa1=10  B_m=10  C_m=1.9  D_m=1  E_m=0.97  fz0=4e+3 N  p_Cx=1.685  p_Dx=[ 1.21 -0.037 ]  p_Ex=[ 0.344 0.095 -0.02 0 ]  p_Kx=[ 21.51 -0.163 0.245 ]  p_Hx=[ -0.002 0.002 ]  p_Vx=[ 0 0 ]  r_e=(t_jantes_av*25.4+2*l_pneu_av*h_broul_av/100)/2 mm  model_compliance=sdl.enum.compliance.on  stiffness=1e+6 N/m  damping=1000 N/(m/s)  model_inertia=sdl.enum.model_inertia.on  inertia=0.12 kg*m^2  initial_velocity=0 rad/s  model_resistance=simscape.enum.onoff.on  resistance_model=sdl.enum.rollingResistanceParameterization.velocity  coeff=0.027*Pe  p_tire=Prar bar  alpha=-0.003  beta=0.76  coeff_a=84e-4  coeff_b=6.2e-4 s/m  coeff_c=1.6e-4 s^2/m^2  v_thr=1e-3 m/s  v_tr_thr=0.1 m/s
  Roue avant droite : sdl_lib/Tires & Vehicles/Tire (Magic Formula)  parameterization=sdl.enum.magic_tire_model.constant  F_z1=3e+3 N  F_x1=3.5e+3 N  kappa1=10  B_m=10  C_m=1.9  D_m=1  E_m=0.97  fz0=4e+3 N  p_Cx=1.685  p_Dx=[ 1.21 -0.037 ]  p_Ex=[ 0.344 0.095 -0.02 0 ]  p_Kx=[ 21.51 -0.163 0.245 ]  p_Hx=[ -0.002 0.002 ]  p_Vx=[ 0 0 ]  r_e=(t_jantes_av*25.4+2*l_pneu_av*h_broul_av/100)/2 mm  model_compliance=sdl.enum.compliance.on  stiffness=1e+6 N/m  damping=1000 N/(m/s)  model_inertia=sdl.enum.model_inertia.on  inertia=0.12 kg*m^2  initial_velocity=0 rad/s  model_resistance=simscape.enum.onoff.on  resistance_model=sdl.enum.rollingResistanceParameterization.velocity  coeff=0.027*Pe  p_tire=Prav bar  alpha=-0.003  beta=0.76  coeff_a=84e-4  coeff_b=6.2e-4 s/m  coeff_c=1.6e-4 s^2/m^2  v_thr=1e-3 m/s  v_tr_thr=0.1 m/s
  Roue avant gauche : sdl_lib/Tires & Vehicles/Tire (Magic Formula)  parameterization=sdl.enum.magic_tire_model.constant  F_z1=3e+3 N  F_x1=3.5e+3 N  kappa1=10  B_m=10  C_m=1.9  D_m=1  E_m=0.97  fz0=4e+3 N  p_Cx=1.685  p_Dx=[ 1.21 -0.037 ]  p_Ex=[ 0.344 0.095 -0.02 0 ]  p_Kx=[ 21.51 -0.163 0.245 ]  p_Hx=[ -0.002 0.002 ]  p_Vx=[ 0 0 ]  r_e=(t_jantes_av*25.4+2*l_pneu_av*h_broul_av/100)/2 mm  model_compliance=sdl.enum.compliance.on  stiffness=1e+6 N/m  damping=1000 N/(m/s)  model_inertia=sdl.enum.model_inertia.on  inertia=0.12 kg*m^2  initial_velocity=0 rad/s  model_resistance=simscape.enum.onoff.on  resistance_model=sdl.enum.rollingResistanceParameterization.velocity  coeff=0.027*Pe  p_tire=Prav bar  alpha=-0.003  beta=0.76  coeff_a=84e-4  coeff_b=6.2e-4 s/m  coeff_c=1.6e-4 s^2/m^2  v_thr=1e-3 m/s  v_tr_thr=0.1 m/s
  Simulink-PS Converter : nesl_utility/Simulink-PS Converter  PhysicalDomain=network_engine_domain  SubClassName=ps_input  LeftPortType=input  RightPortType=output  PseudoPeriodic=off  Frequencies=[]  NoiseDistribution=none  NoiseParameters=[]  Unit=m/s  AffineConversion=off  FilteringAndDerivatives=zero  SimscapeFilterOrder=1  InputFilterTimeConstant=0.001  UdotUserProvided=1
  Simulink-PS Converter1 : nesl_utility/Simulink-PS Converter  PhysicalDomain=network_engine_domain  SubClassName=ps_input  LeftPortType=input  RightPortType=output  PseudoPeriodic=off  Frequencies=[]  NoiseDistribution=none  NoiseParameters=[]  Unit=rad  AffineConversion=off  FilteringAndDerivatives=zero  SimscapeFilterOrder=1  InputFilterTimeConstant=0.001  UdotUserProvided=1
  Simulink-PS Converter2 : nesl_utility/Simulink-PS Converter  PhysicalDomain=network_engine_domain  SubClassName=ps_input  LeftPortType=input  RightPortType=output  PseudoPeriodic=off  Frequencies=[]  NoiseDistribution=none  NoiseParameters=[]  Unit=N  AffineConversion=off  FilteringAndDerivatives=zero  SimscapeFilterOrder=1  InputFilterTimeConstant=0.001  UdotUserProvided=1
  Simulink-PS Converter3 : nesl_utility/Simulink-PS Converter  PhysicalDomain=network_engine_domain  SubClassName=ps_input  LeftPortType=input  RightPortType=output  PseudoPeriodic=off  Frequencies=[]  NoiseDistribution=none  NoiseParameters=[]  Unit=N  AffineConversion=off  FilteringAndDerivatives=zero  SimscapeFilterOrder=1  InputFilterTimeConstant=0.001  UdotUserProvided=1
  Sol : fl_lib/Mechanical/Translational Elements/Mechanical Translational Reference
  Trigonometric Function : Trigonometry  Operator=atan
  Vehicle Body : sdl_lib/Tires & Vehicles/Vehicle Body  mass=M_twizy+M_cond+M_pass+M_Batt kg  n_w=n  x_f=a mm  x_r=b mm  y_c=h mm  mass_var=simscape.enum.onoff.off  g=9.81 m/s^2  liftoff_warning=simscape.enum.onoff.off  area=S m^2  Cd=Cx  rho=1.18 kg/m^3  model_pitch=simscape.enum.onoff.on  inertia=4000 kg*m^2  suspension_model=sdl.enum.linearTLU.linear  k_f=1e4 N/m  b_f=1e4 N/(m/s)  k_r=1e4 N/m  b_r=1e4 N/(m/s)  k_f_TLU=[-2000, -1000, 0, 1000, 2000] N  x_f_TLU=[-.4, -.2, 0, .2, .4] m  b_f_TLU=[-200, -100, 0, 100, 200] N  v_f_TLU=[-4, -2, 0, 2, 4] m/s  k_r_TLU=[-2000, -1000, 0, 1000, 2000] N  x_r_TLU=[-.4, -.2, 0, .2, .4] m  b_r_TLU=[-200, -100, 0, 100, 200] N  v_r_TLU=[-4, -2, 0, 2, 4] m/s  interp_method=simscape.enum.interpolation.linear  extrap_method=simscape.enum.extrapolation.linear  model_hardstop=simscape.enum.onoff.off  upper_bound_f=.25 m  lower_bound_f=-.25 m  stop_k_f=1e6 N/m  stop_b_f=150 N/(m/s)  upper_bound_r=.25 m  lower_bound_r=-.25 m  stop_k_r=1e6 N/m  stop_b_r=150 N/(m/s)  initial_pitch=0 rad  initial_pitch_rate=0 rad/s  v_specify=on  v_priority=High  v=0 m/s  v_nominal_specify=off  v_nominal_unit=m/s  v_nominal_value=1
  Axe roues arrières : PMIOPort  Side=Left
  Bus : Outport  VectorParamsAs1DForOutWhenUnconnected=off
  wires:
  Capteur _meca_translation/1(Out6) -> Bus/1  "Bus_meca_translation"
  Bus Selector/1 -> Gain/1  "<Vent en km/h>"
  PS-Simulink Converter1/1 -> [FN_AV]
  PS-Simulink Converter/1 -> [FN_AR]
  Gain/1 -> Simulink-PS Converter/1
  Gain1/1 -> Trigonometric Function/1
  Trigonometric Function/1 -> Simulink-PS Converter1/1
  Demux/2 -> Simulink-PS Converter2/1
  Forces freinages avant et arrières/1 -> Demux/1
  Demux/1 -> Simulink-PS Converter3/1
  Bus Selector/2 -> Gain1/1  "<Pente en %>"
  Contexte/1 -> Bus Selector/1
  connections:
  Capteur _meca_translation/LConn2 -- Sol/LConn1
  Vehicle Body/LConn1 -- Capteur _meca_translation/RConn1
  Differential/RConn2 -- Roue arriere gauche/LConn2 -- Loaded-Contact Rotational Friction1/RConn1
  Vehicle Body/LConn3 -- Simulink-PS Converter/RConn1
  Vehicle Body/RConn3 -- Simulink-PS Converter1/RConn1
  Roue avant gauche/LConn1 -- PS Gain/RConn1
  Roue arriere gauche/LConn1 -- PS Gain2/RConn1
  Simulink-PS Converter2/RConn1 -- Loaded-Contact Rotational Friction1/LConn1 -- Loaded-Contact Rotational Friction2/LConn1
  Roue avant droite/RConn2 -- Roue avant gauche/RConn2 -- Roue arriere gauche/RConn2 -- Roue arriere droite/RConn2 -- Capteur _meca_translation/LConn1
  Rotational Free End/LConn1 -- Roue avant droite/LConn2 -- Roue avant gauche/LConn2 -- Loaded-Contact Rotational Friction3/RConn1 -- Loaded-Contact Rotational Friction/RConn1
  Roue avant gauche/RConn1 -- PS Terminator/LConn1
  Roue avant droite/RConn1 -- PS Terminator1/LConn1
  Roue arriere gauche/RConn1 -- PS Terminator2/LConn1
  Roue arriere droite/RConn1 -- PS Terminator3/LConn1
  Mechanical Rotational Reference/LConn1 -- Loaded-Contact Rotational Friction/LConn2
  Mechanical Rotational Reference1/LConn1 -- Loaded-Contact Rotational Friction1/LConn2
  PS Terminator4/LConn1 -- Vehicle Body/LConn2
  Simulink-PS Converter3/RConn1 -- Loaded-Contact Rotational Friction3/LConn1 -- Loaded-Contact Rotational Friction/LConn1
  Differential/LConn1 -- Axe roues arrières/RConn1
  Differential/RConn1 -- Roue arriere droite/LConn2 -- Loaded-Contact Rotational Friction2/RConn1
  Mechanical Rotational Reference2/LConn1 -- Loaded-Contact Rotational Friction3/LConn2
  Loaded-Contact Rotational Friction2/LConn2 -- Mechanical Rotational Reference3/LConn1
  Vehicle Body/RConn2 -- PS-Simulink Converter1/LConn1 -- PS Gain1/LConn1 -- PS Gain/LConn1
  Roue avant droite/LConn1 -- PS Gain1/RConn1
  PS-Simulink Converter/LConn1 -- Vehicle Body/RConn1 -- PS Gain3/LConn1 -- PS Gain2/LConn1
  Roue arriere droite/LConn1 -- PS Gain3/RConn1

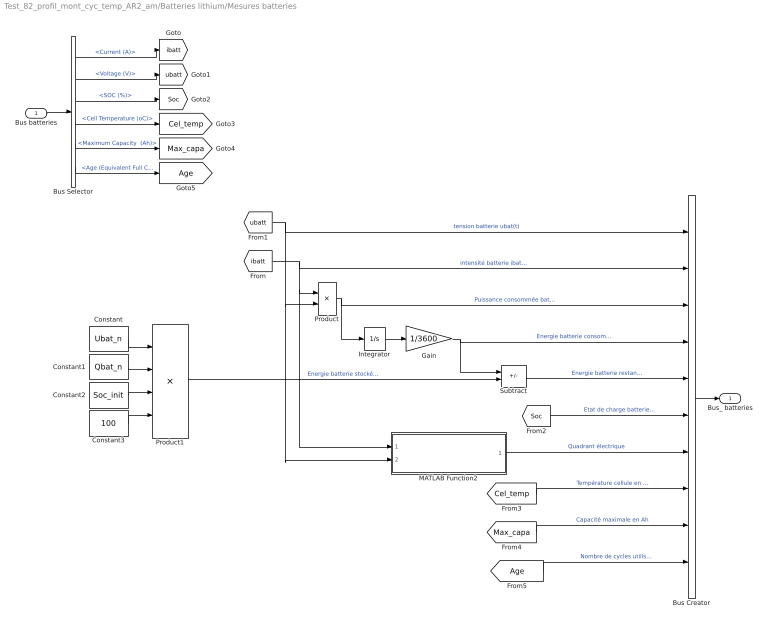
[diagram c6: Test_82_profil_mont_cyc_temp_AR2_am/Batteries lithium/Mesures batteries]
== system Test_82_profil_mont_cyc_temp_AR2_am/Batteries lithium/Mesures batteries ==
  Bus batteries : Inport
  Bus Creator : BusCreator  Inputs=10
  Bus Selector : BusSelector  OutputSignals="Current (A),Voltage (V),SOC (%),Cell Temperature (oC),Maximum Capacity  (Ah),Age (Equivalent Full Cycles)"
  Constant : Constant  Value=Ubat_n
  Constant1 : Constant  Value=Qbat_n
  Constant2 : Constant  Value=Soc_init
  Constant3 : Constant  Value=100
  Gain : Gain  Gain=1/3600
  Integrator : Integrator
  MATLAB Function2 : MATLAB Function  TreatAsAtomicUnit=on
  Product : Product
  Product1 : Product  Inputs=***/
  Subtract : Sum  Inputs=-+
  Bus_ batteries : Outport  VectorParamsAs1DForOutWhenUnconnected=off
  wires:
  Bus batteries/1 -> Bus Selector/1
  Product/1 -> Bus Creator/3, Integrator/1  "Puissance consommée batterie pbat(t) en W"
  Bus Creator/1 -> Bus_ batteries/1
  Integrator/1 -> Gain/1
  Gain/1 -> Bus Creator/4, Subtract/1  "Energie batterie consommée wbat_cons(t) en Wh"
  [ibatt] -> Bus Creator/2, MATLAB Function2/1(I_bat), Product/1  "intensité batterie ibat(t)"
  Bus Selector/1 -> [ibatt]  "<Current (A)>"
  Bus Selector/2 -> [ubatt]  "<Voltage (V)>"
  [ubatt] -> MATLAB Function2/2(U_bat), Product/2, Bus Creator/1  "tension batterie ubat(t)"
  Bus Selector/3 -> [Soc]  "<SOC (%)>"
  [Soc] -> Bus Creator/6  "Etat de charge batterie soc(t) en %"
  MATLAB Function2/1(Quadrant_elec) -> Bus Creator/7  "Quadrant électrique"
  Constant/1 -> Product1/1
  Constant1/1 -> Product1/2
  Constant2/1 -> Product1/3
  Constant3/1 -> Product1/4
  Subtract/1 -> Bus Creator/5  "Energie batterie restante wbat_rest(t) en Wh"
  Product1/1 -> Subtract/2  "Energie batterie stockée wstock_batt(t) en Wh"
  Bus Selector/4 -> [Cel_temp]  "<Cell Temperature (oC)>"
  Bus Selector/5 -> [Max_capa]  "<Maximum Capacity  (Ah)>"
  Bus Selector/6 -> [Age]  "<Age (Equivalent Full Cycles)>"
  [Cel_temp] -> Bus Creator/8  "Température cellule en °C"
  [Max_capa] -> Bus Creator/9  "Capacité maximale en Ah"
  [Age] -> Bus Creator/10  "Nombre de cycles utilisés"

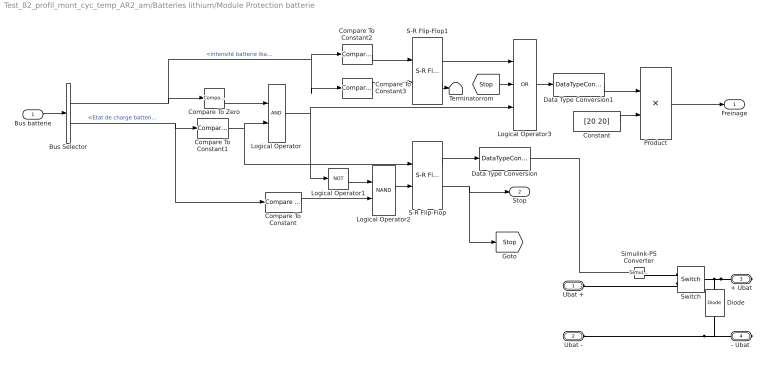
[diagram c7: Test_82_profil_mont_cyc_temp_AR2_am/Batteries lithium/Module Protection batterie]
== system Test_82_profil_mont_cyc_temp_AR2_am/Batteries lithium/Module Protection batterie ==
  Bus batterie : Inport
  Bus Selector : BusSelector  OutputSignals=intensité batterie ibat(t),Etat de charge batterie soc(t) en %
  Compare To Constant : simulink/Logic and Bit Operations/Compare To Constant  relop=>  const=Soc_min  OutDataTypeStr=boolean
  Compare To Constant1 : simulink/Logic and Bit Operations/Compare To Constant  relop=>=  const=100  OutDataTypeStr=boolean
  Compare To Constant2 : simulink/Logic and Bit Operations/Compare To Constant  relop=<=  const=-205  OutDataTypeStr=boolean
  Compare To Constant3 : simulink/Logic and Bit Operations/Compare To Constant  relop=>=  const=-185  OutDataTypeStr=boolean
  Compare To Zero : simulink/Logic and Bit Operations/Compare To Zero  relop=<  OutDataTypeStr=boolean
  Constant : Constant  Value=[20 20]
  Data Type Conversion : DataTypeConversion  OutDataTypeStr=double
  Data Type Conversion1 : DataTypeConversion  OutDataTypeStr=double
  Diode : fl_lib/Electrical/Electrical Elements/Diode  Vf=0.6 V  Ron=0.3 Ohm  Goff=1e-8 1/Ohm  i_specify=off  i_priority=None  i=0 A  i_nominal_specify=off  i_nominal_unit=A  i_nominal_value=1  v_specify=off  v_priority=None  v=0 V  v_nominal_specify=off  v_nominal_unit=V  v_nominal_value=1
  Logical Operator : Logic  AllPortsSameDT=off  OutDataTypeStr=boolean
  Logical Operator1 : Logic  Operator=NOT  AllPortsSameDT=off  OutDataTypeStr=boolean
  Logical Operator2 : Logic  Operator=NAND  AllPortsSameDT=off  OutDataTypeStr=boolean
  Logical Operator3 : Logic  Operator=OR  Inputs=3  AllPortsSameDT=off  OutDataTypeStr=boolean
  Product : Product
  S-R Flip-Flop : simulink_extras/Flip Flops/S-R Flip-Flop  initial_condition=1
  S-R Flip-Flop1 : simulink_extras/Flip Flops/S-R Flip-Flop  initial_condition=1
  Simulink-PS Converter : nesl_utility/Simulink-PS Converter  PhysicalDomain=network_engine_domain  SubClassName=ps_input  LeftPortType=input  RightPortType=output  PseudoPeriodic=off  Frequencies=[]  NoiseDistribution=none  NoiseParameters=[]  Unit=1  AffineConversion=off  FilteringAndDerivatives=provide  SimscapeFilterOrder=1  InputFilterTimeConstant=0.001  UdotUserProvided=0
  Switch : fl_lib/Electrical/Electrical Elements/Switch  R_closed=0.01 Ohm  G_open=1e-8 1/Ohm  Threshold=0.5  i_specify=off  i_priority=None  i=0 A  i_nominal_specify=off  i_nominal_unit=A  i_nominal_value=1  v_specify=off  v_priority=None  v=0 V  v_nominal_specify=off  v_nominal_unit=V  v_nominal_value=1
  Terminator : Terminator
  Ubat + : PMIOPort  Side=Left
  Ubat - : PMIOPort  Port=2  Side=Left
  + Ubat : PMIOPort  Port=3  Side=Right
  "- Ubat " : PMIOPort  Port=4  Side=Right
  Freinage : Outport  VectorParamsAs1DForOutWhenUnconnected=off
  Stop : Outport  Port=2  VectorParamsAs1DForOutWhenUnconnected=off
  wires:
  Bus Selector/2 -> Compare To Constant/1, Compare To Constant1/1  "<Etat de charge batterie soc(t) en %>"
  Compare To Constant/1 -> Logical Operator2/2
  Compare To Constant1/1 -> S-R Flip-Flop/1, Logical Operator/2
  Bus Selector/1 -> Compare To Constant3/1, Compare To Constant2/1, Compare To Zero/1  "<intensité batterie ibat(t)>"
  Compare To Zero/1 -> Logical Operator/1
  Logical Operator/1 -> Logical Operator1/1, Logical Operator3/3
  Data Type Conversion1/1 -> Product/1
  Logical Operator1/1 -> Logical Operator2/1
  Logical Operator2/1 -> S-R Flip-Flop/2
  Product/1 -> Freinage/1
  Constant/1 -> Product/2
  Bus batterie/1 -> Bus Selector/1
  Data Type Conversion/1 -> Simulink-PS Converter/1
  S-R Flip-Flop/2 -> [Stop], Stop/1
  S-R Flip-Flop/1 -> Data Type Conversion/1
  Logical Operator3/1 -> Data Type Conversion1/1
  [Stop] -> Logical Operator3/2
  Compare To Constant2/1 -> S-R Flip-Flop1/1
  S-R Flip-Flop1/1 -> Logical Operator3/1
  Compare To Constant3/1 -> S-R Flip-Flop1/2
  S-R Flip-Flop1/2 -> Terminator/1
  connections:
  + Ubat/RConn1 -- Switch/LConn1 -- Diode/RConn1
  Simulink-PS Converter/RConn1 -- Switch/RConn1
  Ubat -/RConn1 -- "- Ubat "/RConn1 -- Diode/LConn1
  Switch/RConn2 -- Ubat +/RConn1

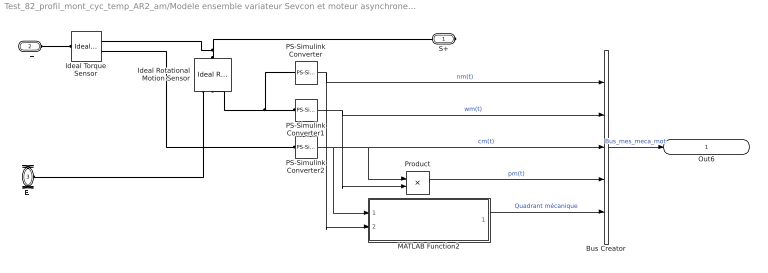
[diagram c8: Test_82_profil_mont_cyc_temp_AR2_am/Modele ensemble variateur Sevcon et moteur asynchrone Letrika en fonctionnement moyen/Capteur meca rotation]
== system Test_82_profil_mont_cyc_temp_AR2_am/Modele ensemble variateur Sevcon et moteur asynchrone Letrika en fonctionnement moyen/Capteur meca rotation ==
  Bus Creator : BusCreator  Inputs=5
  Ideal Rotational Motion Sensor : fl_lib/Mechanical/Mechanical Sensors/Ideal Rotational Motion Sensor  wrap_angle=simscape.enum.onoff.off  offset=0 rad
  Ideal Torque Sensor : fl_lib/Mechanical/Mechanical Sensors/Ideal Torque Sensor
  MATLAB Function2 : MATLAB Function  TreatAsAtomicUnit=on
  PS-Simulink Converter : nesl_utility/PS-Simulink Converter  PhysicalDomain=network_engine_domain  SubClassName=ps_output  LeftPortType=input  RightPortType=output  PseudoPeriodic=off  Frequencies=[]  Unit=rpm  AffineConversion=off
  PS-Simulink Converter1 : nesl_utility/PS-Simulink Converter  PhysicalDomain=network_engine_domain  SubClassName=ps_output  LeftPortType=input  RightPortType=output  PseudoPeriodic=off  Frequencies=[]  Unit=rad/s  AffineConversion=off
  PS-Simulink Converter2 : nesl_utility/PS-Simulink Converter  PhysicalDomain=network_engine_domain  SubClassName=ps_output  LeftPortType=input  RightPortType=output  PseudoPeriodic=off  Frequencies=[]  Unit=N*m  AffineConversion=off
  Product : Product
  S+ : PMIOPort  Side=Right
  E+ : PMIOPort  Port=2  Side=Left
  E- : PMIOPort  Port=3  Side=Left
  Out6 : Outport  VectorParamsAs1DForOutWhenUnconnected=off
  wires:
  PS-Simulink Converter/1 -> MATLAB Function2/2(Nm), Bus Creator/1  "nm(t)"
  Product/1 -> Bus Creator/4  "pm(t)"
  Bus Creator/1 -> Out6/1  "Bus_mes_meca_mot"
  PS-Simulink Converter1/1 -> Product/2, Bus Creator/2  "wm(t)"
  PS-Simulink Converter2/1 -> MATLAB Function2/1(Cm), Product/1, Bus Creator/3  "cm(t)"
  MATLAB Function2/1(Quadrant_meca) -> Bus Creator/5  "Quadrant mécanique"
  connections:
  PS-Simulink Converter2/LConn1 -- Ideal Torque Sensor/RConn2
  Ideal Rotational Motion Sensor/LConn1 -- S+/RConn1 -- Ideal Torque Sensor/RConn1
  PS-Simulink Converter1/LConn1 -- Ideal Rotational Motion Sensor/RConn2 -- PS-Simulink Converter/LConn1
  Ideal Torque Sensor/LConn1 -- E+/RConn1
  Ideal Rotational Motion Sensor/RConn1 -- E-/RConn1
